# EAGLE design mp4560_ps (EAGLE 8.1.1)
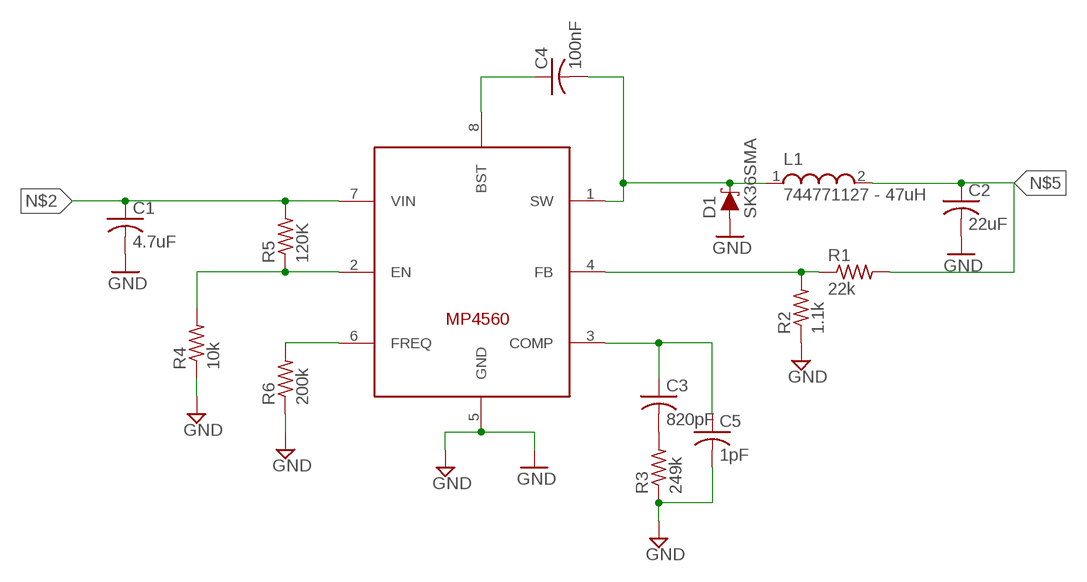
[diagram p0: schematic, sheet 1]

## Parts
C1  4.7uF  C-USC1210  [C1210]
C2  22uF  C-USC1210  [C1210]
C3  820pF  C-USC0805  [C0805]
C4  100nF  C-USC0805  [C0805]
C5  1pF  C-USC0805  [C0805]
D1  SK36SMA  DIODE-SCHOTTKY-B340A  [SMA-DIODE]
L1  744771127 - 47uH  WE-PD_1260/1245/1280/1210  [WE-PD_1260/1245/1280/1210]
R1  22k  R-US_R0805  [R0805]
R2  1.1k  R-US_R0805  [R0805]
R3  249k  R-US_R0805  [R0805]
R4  10k  R-US_R0805  [R0805]
R5  120K  R-US_R0805  [R0805]
R6  200k  R-US_R0805  [R0805]
U$1  MP4560  [SOIC8]

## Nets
GND: C1.2 C2.2 C5.2 D1.A R2.1 R3.1 R4.1 R6.1 U$1.5(GND)
N$1: R4.2 R5.1 U$1.2(EN)
N$2: C1.1 R5.2 U$1.7(VIN)
N$3: R6.2 U$1.6(FREQ)
N$4: R1.1 R2.2 U$1.4(FB)
N$5: C2.1 L1.2 R1.2
N$6: C4.1 U$1.8(BST)
N$8: C4.2 D1.C L1.1 U$1.1(SW)
N$9: C3.2 R3.2
N$10: C3.1 C5.1 U$1.3(COMP)

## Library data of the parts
C1-C5 = adafruit:C-US: CAPACITOR, American symbol
D1 = SparkFun-DiscreteSemi:DIODE-SCHOTTKY: Schottky diode; PROD_ID: DIO-09886; VALUE: 3A/40V/500mV
L1 = EAGLE-POWER_MAGNETICS-rev17a:WE-PD: SMD Shielded Power Inductor
R1-R6 = adafruit:R-US_: RESISTOR, American symbol
U$1 = so8-0005:MP4560

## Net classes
0 default: clearance 0.254 mm

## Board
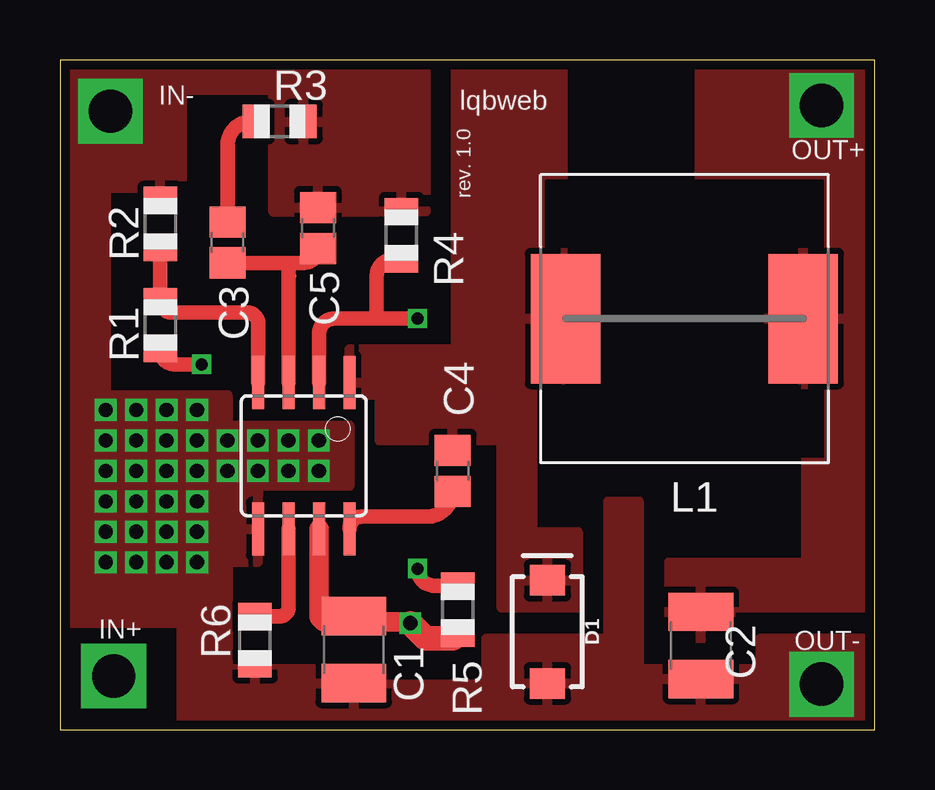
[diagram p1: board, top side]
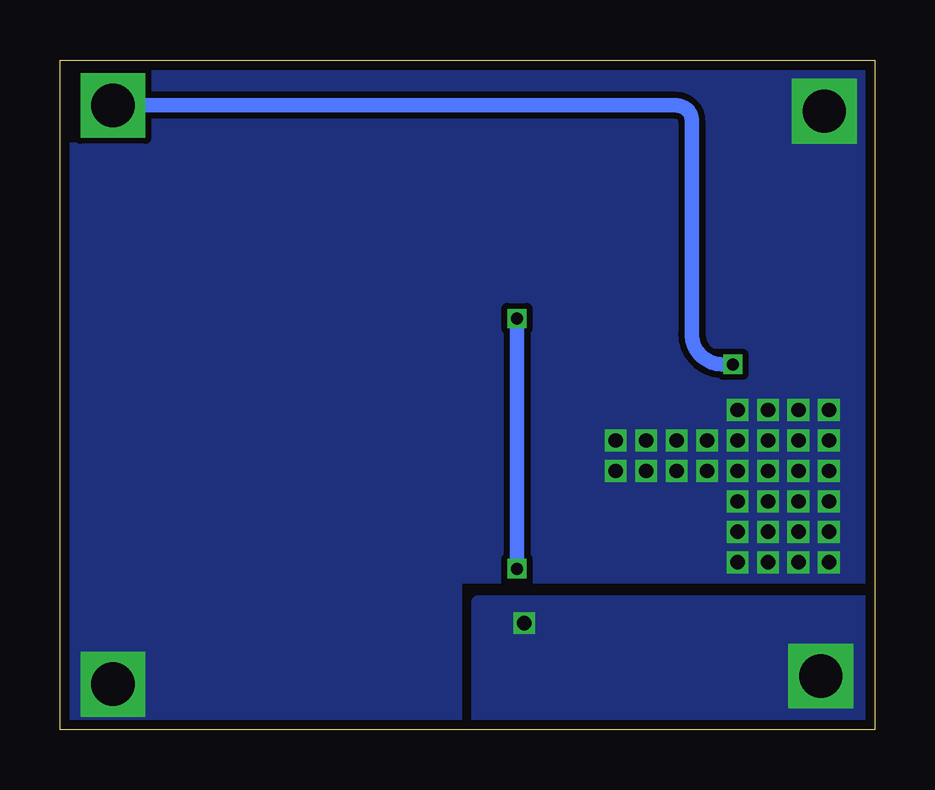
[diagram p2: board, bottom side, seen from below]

Size 33.96 x 27.93 mm. Coordinates in mm from the lower left corner, seen from the top.
Outline: 0,0 33.96,0 33.96,27.93 0,27.93 0,0
Copper layers (1*16): Top 0.035mm / dielectric 1.5mm / Bottom 0.035mm
Design rules "NOA Eagle Rule 2016-06-12": minimum track width 6mil, minimum drill 0.3mm, track to track 6mil, track to pad 6mil, pad to pad 6mil, via to via 6mil, smd to smd 0mil, copper to edge 0.4mm, drill to drill 10mil, minimum pad ring 10mil, minimum via ring 6mil, stop-mask expansion 2mil, vias tented up to drill 25mil, thermal gap 10mil

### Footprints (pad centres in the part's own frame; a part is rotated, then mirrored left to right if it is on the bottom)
C1210 = smd 1.6 x 2.7: 1 -1.4,0; 2 1.4,0
C0805 = smd 1.3 x 1.5: 1 -0.85,0; 2 0.85,0
SMA-DIODE = smd 1.27 x 1.47: A -2.15,0; C 2.15,0
WE-PD_1260/1245/1280/1210 = smd 2.9 x 5.4: 1 -4.95,0; 2 4.95,0
R0805 = smd 1.1 x 1.4: 1 -1,0; 2 1,0
SOIC8 = smd 0.5 x 2.2: 1 -1.905,-3.048; 2 -0.645,-3.048; 3 0.625,-3.048; 4 1.895,-3.048; 5 1.905,3.048; 6 0.635,3.048; 7 -0.635,3.048; 8 -1.905,3.048

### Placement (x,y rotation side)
C1  12.25,3.35 270 top
C2  26.72,3.52 270 top
C3  6.99,20.32 90 top
C4  16.37,10.79 90 top
C5  10.76,20.92 90 top
D1  20.32,4.09 90 top
L1  26.04,17.14 0 top
R1  4.18,16.88 270 top
R2  4.18,21.09 270 top
R3  9.15,25.36 180 top
R4  14.23,20.62 270 top
R5  16.58,5.01 270 top
R6  8.13,3.74 90 top
U$1  10.16,11.43 180 top

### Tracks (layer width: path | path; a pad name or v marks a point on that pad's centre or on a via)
GND  (via drill 0.6, 1.8)
  other vias: 4.45,10.79 3.17,10.79 1.91,10.79 5.71,10.79 1.91,12.06 4.45,12.06 3.17,12.06 5.71,12.06 6.99,12.06 8.26,12.06 9.53,12.06 10.79,12.06 10.79,10.79 9.53,10.79 8.26,10.79 6.99,10.79 1.91,9.53 3.17,9.53 4.45,9.53 5.71,9.53 1.91,8.26 3.17,8.26 4.45,8.26 5.71,8.26 1.91,6.99 3.17,6.99 4.45,6.99 5.71,6.99 1.91,13.34 3.17,13.34 4.45,13.34 5.71,13.34 31.75,1.91 2.1,25.8
  pour Top: 15.24,21.59 8.89,21.59 8.89,26.67 5.08,26.67 5.08,22.59 1.91,22.59 1.91,13.97 6.99,13.97 6.99,12.7 12.06,12.7 12.06,10.16 8.26,10.16 8.26,6.99 6.99,6.99 6.99,2.54 13.34,2.54 13.34,1.91 17.78,1.91 17.78,3.81 22.86,3.81 22.86,9.53 24.13,9.53 24.13,2.54 29.21,2.54 29.21,3.81 34.29,3.81 34.29,0 5.08,0 5.08,4.45 0,4.45 0,29.21 15.24,29.21
  pour Bottom: -0.6,29.1 -0.6,6.6 -0.6,6.3 17.4,6.3 17.4,-0.6 35.1,-0.6 35.1,29.1
N$1  (via drill 0.5)
  Top 0.406: R4.2 13.92,19.62
  Top 0.61: U$1.2 10.8,16.52 arc-90 11.43,17.14 13.2,17.14 | 13.2,17.14 v14.9,17.14 | 13.92,19.62 arc90 13.2,18.9 13.2,17.14 | v14.9,6.72 arc90 15.62,6.01 R5.1
  Bottom 0.61: v14.9,17.14 v14.9,6.72
N$2  (via drill 0.6, 1.8)
  Top 0.406: 14.55,4.5 arc-90 v14.61,4.45 | U$1.7 arc90 U$1.7 | 12.45,4.75 arc-90 12.7,4.5
  Top 0.61: R5.2 arc-90 16.38,3.81
  Top 0.813: 14.55,4.5 12.7,4.5 11.1,4.5 arc-90 10.8,4.8 U$1.7 | C1.1 12.45,4.75
  Top 1.016: 16.38,3.81 15.24,3.81 v14.61,4.45
  other vias: 2.24,2.24
  pour Bottom: 0,5.31 16.51,5.31 16.51,0 0,0
N$3
  Top 0.61: U$1.6 9.53,5.08 arc-90 9.19,4.74 R6.2
N$4
  Top 0.61: R2.2 R1.1 arc90 4.66,17.4 7.8,17.4 arc-90 8.27,16.93 U$1.4
N$5  (via drill 0.5, 1.8)
  Top 0.406: 31.75,25.4 v31.75,26.04 31.75,26.67
  Top 0.61: R1.2 arc90 4.75,15.24 v5.91,15.24
  Bottom 0.61: v31.75,26.04 8.26,26.04 arc90 7.62,25.4 7.62,16.51 arc-90 6.35,15.24 v5.91,15.24
  pour Top: 27.94,3.81 25.4,3.81 25.4,6.99 31.11,6.99 31.11,14.61 26.67,14.61 26.67,28.57 33.66,28.57 33.66,5.08 27.94,5.08
N$6
  Top 0.61: 16.51,10.16 16.51,10.09 arc-90 C4.1 arc-90 15.31,8.89 12.57,8.89 arc90 U$1.8
N$8
  pour Top: 12.06,13.97 12.06,15.88 16.51,15.88 16.51,27.94 20.95,27.94 20.95,14.61 19.68,14.61 19.68,8.26 21.59,8.26 21.59,5.08 18.41,5.08 18.41,12.06 13.34,12.06 13.34,13.97
N$9
  Top 0.61: R3.2 arc90 6.99,24.5 C3.2
N$10
  Top 0.406: 9.65,18.92 arc-90 9.53,19.05
  Top 0.61: 8.89,19.47 9.53,19.47 9.53,19.05 9.53,14.49 arc90 U$1.3 | 8.89,19.47 C3.1 | 8.89,19.47 10.16,19.47 arc90 C5.1

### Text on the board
tPlace: lqbweb | IN- | rev. 1.0 | OUT+ | IN+ | OUT-

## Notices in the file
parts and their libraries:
SparkFun-DiscreteSemi: Licensing: Creative Commons ShareAlike 4.0 International - https://creativecommons.org/licenses/by-sa/4.0
EAGLE-POWER_MAGNETICS-rev17a: Copyright: Würth Elektronik
